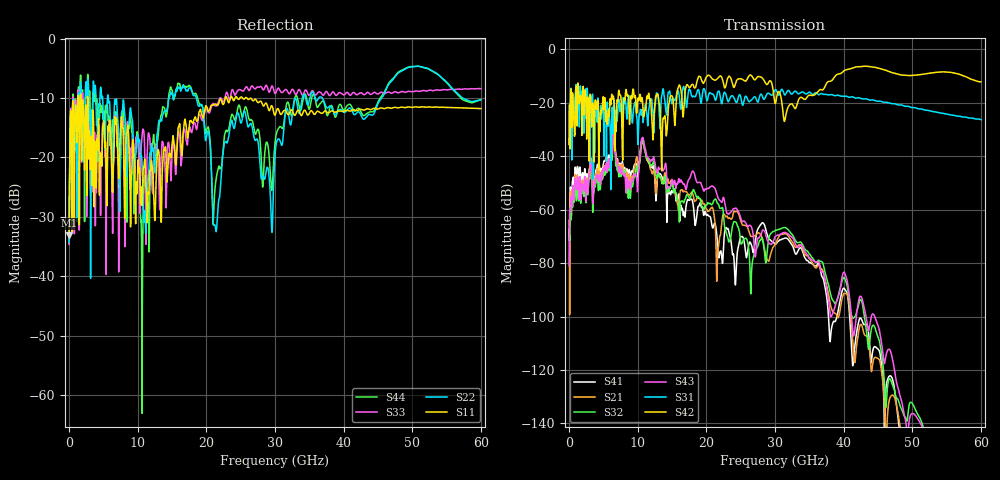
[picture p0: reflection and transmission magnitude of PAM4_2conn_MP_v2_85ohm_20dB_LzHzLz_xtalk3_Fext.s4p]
! Info: Touchstone file created by Circ.  Input file=FAB50GbE_2conn_Midplane_Examax_Topo2_v2_85ohm_20dB_LzHzLz.circ
# Hz S RI R 50
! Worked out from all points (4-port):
!   6000 points, 10 MHz to 60 GHz, reference 50 ohm
!   strongest paths, dB at 10 MHz, 15.01 GHz, 30.01 GHz, 45.01 GHz, 60 GHz:
!     S42: -35.6, -17.4, -20.2, -7.0, -12.1
!     S31: -35.4, -20.0, -15.1, -19.3, -26.3
!     S43: -80.9, -48.6, -70.2, -103.4, -156.5
!     S32: -68.0, -49.2, -67.7, -107.6, -152.0
!     S21: -64.0, -50.1, -72.9, -115.7, -159.2
!     S41: -67.5, -53.0, -72.6, -112.2, -175.8
!   lowest |S11| = -33.1 dB at 10 MHz (marker M1), VSWR 1.05, Z = 52 - j1.12 ohm
!   |S11| at or under -10 dB: start of sweep to 1.305 GHz; 2.75 GHz to 22.78 GHz (20.03 GHz wide, 157 % of centre); 25.91 GHz to end of sweep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
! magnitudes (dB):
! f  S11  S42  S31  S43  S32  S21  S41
! 10 MHz  -33.1  -35.6  -35.4  -80.9  -68.0  -64.0  -67.5
! 1.09 GHz  -14.3  -15.3  -15.5  -52.3  -56.3  -53.7  -49.8
! 10.75 GHz  -23.5  -21.0  -26.5  -32.9  -34.1  -34.8  -33.6
! 14.8 GHz  -20.0  -17.3  -18.1  -51.2  -51.5  -49.3  -54.4
! 22.12 GHz  -10.2  -10.0  -18.9  -56.9  -59.5  -68.4  -75.5
! 26.57 GHz  -10.1  -9.8  -18.9  -66.5  -84.3  -70.0  -73.1
! 60 GHz  -11.8  -12.1  -26.3  -156.5  -152.0  -159.2  -175.8
